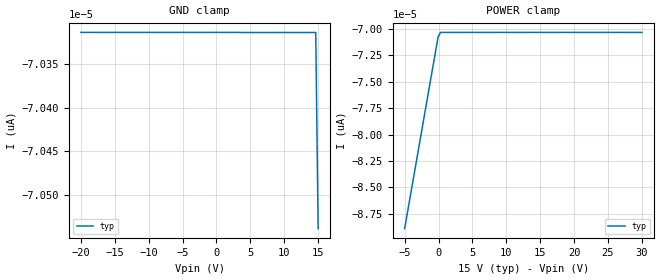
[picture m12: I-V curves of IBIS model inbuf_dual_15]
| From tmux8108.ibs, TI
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| inbuf_dual_15
[Model]   inbuf_dual_15
Model_type   Input
Vinl = 1.3
Vinh = 0.8
|   typ   min   max
C_comp   4.014581e-13   NA   NA
[Voltage Range]   15   NA   NA
[Temperature Range]   27   NA   NA
[Power Clamp Reference]   15   NA   NA
[GND Clamp Reference]   0   NA   NA
[GND Clamp]
|   Voltage   I(typ)   I(min)   I(max)
-20V      -70.31pA   NA         NA
3.333V    -70.31pA   NA         NA
14.65V    -70.31pA   NA         NA
15V       -70.54pA   NA         NA
[POWER Clamp]
|   Voltage   I(typ)   I(min)   I(max)
-5V       -88.91pA   NA         NA
-50.5mV   -70.7pA    NA         NA
303mV     -70.31pA   NA         NA
30V       -70.31pA   NA         NA
